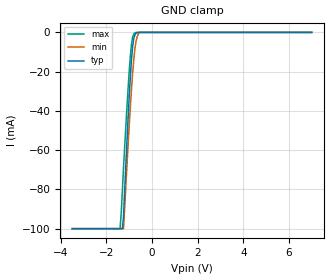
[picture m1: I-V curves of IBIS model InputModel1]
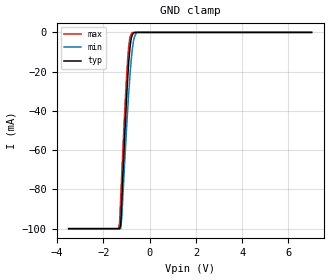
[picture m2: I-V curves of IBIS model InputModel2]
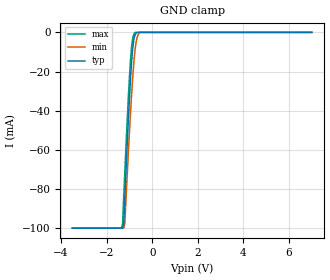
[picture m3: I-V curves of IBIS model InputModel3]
[IBIS Ver]   2.1
[File name]   e_002bl3.ibs   | e_= TSOP, f002bl= abbr chip name, 3= 3.3V Vcc
[File Rev]   2.00
[Date]   13-March-1996
[Source]   File generated from lab measurements at Intel Corporation
[Notes]   Rev 2.00 All data was replaced by actual measurements
   performed in a lab.
[Disclaimer] INTEL DEVELOPER'S SOFTWARE LICENSE AGREEMENT
| BY USING THIS SOFTWARE, YOU ARE AGREEING TO BE BOUND
| BY THE TERMS OFTHIS AGREEMENT.  DO NOT USE THE SOFTWARE
| UNTIL YOU HAVE CAREFULLY READAND AGREED TO THE FOLLOWING
| TERMS AND CONDITIONS.  IF YOU DO NOT AGREETO THE TERMS
| OF THIS AGREEMENT, PROMPTLY RETURN THE SOFTWARE PACKAGE
| ANDANY ACCOMPANYING ITEMS.
| IF YOU USE THIS SOFTWARE, YOU WILL BE BOUND BY THE TERMS
| OF THIS AGREEMENT
| LICENSE: Intel Corporation ("Intel") grants you the non-exclusive right
| to use the enclosed software program ("Software").  You will not use,
| copy, modify, rent, sell or transfer the Software or any portion
| thereof, except as provided in this Agreement.
| System OEM Developers may:
| 1.   Copy the Software for support, backup or archival purposes;
| 2.   Install, use, or distribute Intel owned Software in object code
|   only;
| 3.   Modify and/or use Software source code that Intel directly makes
|   available to you as an OEM Developer;
| 4.   Install, use, modify, distribute, and/or make or have made
|   derivatives ("Derivatives") of Intel owned Software under the
|   terms and conditions in this Agreement, ONLY if you are a System
|   OEM Developer and NOT an end-user.
| RESTRICTIONS:
| YOU WILL NOT:
| 1.   Copy the Software, in whole or in part, except as provided for
|   in this Agreement;
| 2.   Decompile or reverse engineer any Software provided in object
|   code format;
| 3.   Distribute any Software or Derivative code to any end-users,
|   unless approved by Intel in a prior writing.
| TRANSFER: You may transfer the Software to another OEM
| Developer if thereceiving party agrees to the terms of this
| Agreement at the sole risk of any receiving party.
| OWNERSHIP AND COPYRIGHT OF SOFTWARE:
| Title to the Software and all copies thereof remain with Intel
| or its vendors.  The Software iscopyrighted and is protected by
| United States and international copyright laws.  You will not
| remove the copyright notice from the Software.  You agree to
| prevent any unauthorized copying of the Software.
| DERIVATIVE WORK: OEM Developers that make or have made
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[Copyright]   Copyright 1996, Intel Corporation, All Rights Reserved
[Component]   E28F002BL   | 40-lead TSOP package, 28F002BL
[Manufacturer]  Intel   | Boot Block (tm)
|   | operating in 3.3V Vcc range
[Package]
| The following values apply for the Alloy-42 leadframe.
|Variable   typ   min   max
R_pkg   135m   126m   144m
L_pkg   3.95nH   3.62nH   4.28nH
C_pkg   0.39pF   0.38pF   0.40pF
|***********************Pin Definition********************************
[Pin]   signal_name   model_name   R_pin   L_pin   C_pin
  1   A16   InputModel2
  2   A15   InputModel1
  3   A14   InputModel1
  4   A13   InputModel1
  5   A12   InputModel1
  6   A11   InputModel1
  7   A9   InputModel1
  8   A8   InputModel1
  9   WE#   InputModel5
 10   RP#   InputModel3
 11   VPP   POWER
 12   DU   InputModel6
 13   NC   InputModel1
 14   A7   InputModel1
 15   A6   InputModel1
 16   A5   InputModel1
 17   A4   InputModel1
 18   A3   InputModel1
 19   A2   InputModel1
 20   A1   InputModel1
 21   A0   InputModel2
 22   CE#   InputModel2
 23   GND   GND
 24   OE#   InputModel4
 25   DQ0   InputOutput
 26   DQ1   InputOutput
 27   DQ2   InputOutput
 28   DQ3   InputOutput
 29   NC   InputModel2
 30   VCC   POWER
 31   VCC   POWER
 32   DQ4   InputOutput
 33   DQ5   InputOutput
 34   DQ6   InputOutput
 35   DQ7   InputOutput
 36   A10   InputModel1
 37   NC   InputModel6
 38   NC   InputModel6
 39   GND   GND
 40   A17   InputModel1
|***********************Input Model 6******************************
[Model]   InputModel6
Model_type   Input
|   Model for  DU & NC pins, excluding Pin #13.
Vinl = 0.8V
Vinh = 2.0V
|Variable   Typ   Min   Max
C_comp   5.61p   NA   7.6p
[Voltage Range]   3.3V   3.0V   3.6V
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| Models and submodels in the file (7): InputModel1 (Input), InputModel2 (Input), InputModel3 (Input), InputModel4 (Input), InputModel5 (Input), InputModel6 (Input), InputOutput (I/O)
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|*********************Input Model 1************************************
[Model]   InputModel1
Model_type   Input
|   Model for A[15:1] A[17] & NC (pin 13).
Vinl = 0.8V
Vinh = 2.0V
|Variable   Typ   Min   Max
C_comp   5.61p   NA   7.6p
[Voltage Range]   3.3V   3.0V   3.6V
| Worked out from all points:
|   GND clamp passes 1 mA (typ) near -0.74 V on its own axis
[GND_clamp]
|Voltage  I(typ)   I(min)   I(max)
-3.5V     -100mA     -100mA     -100mA
-1.4V     -100mA     -100mA     -100mA
-1.35V    -100mA     -100mA     -92.06mA
-1.3V     -100mA     -100mA     -81.04mA
-1.25V    -94.05mA   -100mA     -69.23mA
-1.1V     -55.84mA   -68.26mA   -38.39mA
-1V       -32.84mA   -47.78mA   -19.9mA
-900mV    -13.97mA   -29.09mA   -6.016mA
-800mV    -3.185mA   -14.07mA   -792.3uA
-700mV    -426.8uA   -4.481mA   0A
-550mV    0A         0A         0A
7V        0A         0A         0A
[Power_clamp]
| Input buffer circuits of this product do not intrinsically
| require a [Power_clamp] definition.  This zero current
| [Power_clamp] table is provided for the compatibility with
| some IBIS parsers.
|Voltage  I(typ)   I(min)   I(max)
-3.3V     0A         0A         0A
0V        0A         0A         0A
3.3V      0A         0A         0A
7V        0A         0A         0A
|*********************Input Model 2******************************
[Model]   InputModel2
Model_type   Input
|   Model for A[0], A[16] & CE# pins.
Vinl = 0.8V
Vinh = 2.0V
|Variable   Typ   Min   Max
C_comp   5.61p   NA   7.6p
[Voltage Range]   3.3V   3.0V   3.6V
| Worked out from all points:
|   GND clamp passes 1 mA (typ) near -0.74 V on its own axis
[GND_clamp]
|Voltage  I(typ)   I(min)   I(max)
-3.5V     -100mA     -100mA     -100mA
-1.35V    -100mA     -100mA     -100mA
-1.3V     -100mA     -100mA     -97.31mA
-1.25V    -97.98mA   -100mA     -83.77mA
-1.2V     -84.29mA   -93.56mA   -70.52mA
-1.05V    -45.71mA   -60.05mA   -33.65mA
-950mV    -23.43mA   -39.44mA   -13.59mA
-850mV    -7.586mA   -21.73mA   -2.468mA
-750mV    -1.17mA    -8.517mA   0A
-650mV    0A         -2.085mA   0A
-550mV    0A         0A         0A
7V        0A         0A         0A
[Power_clamp]
| Input buffer circuits of this product do not intrinsically
| require a [Power_clamp] definition.  This zero current
| [Power_clamp] table is provided for the compatibility with
| some IBIS parsers.
|Voltage  I(typ)   I(min)   I(max)
-3.3V     0A         0A         0A
0V        0A         0A         0A
3.3V      0A         0A         0A
7V        0A         0A         0A
|***********************Input Model 3******************************
[Model]   InputModel3
Model_type   Input
|   Model for RP# pin.
Vinl = 0.8V
Vinh = 2.0V
|Variable   Typ   Min   Max
C_comp   5.61p   NA   7.6p
[Voltage Range]   3.3V   3.0V   3.6V
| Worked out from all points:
|   GND clamp passes 1 mA (typ) near -0.74 V on its own axis
[GND_clamp]
|Voltage  I(typ)   I(min)   I(max)
-3.5V     -100mA     -100mA     -100mA
-1.35V    -100mA     -100mA     -100mA
-1.3V     -100mA     -100mA     -97.77mA
-1.25V    -97.89mA   -100mA     -84.11mA
-1.2V     -84.17mA   -97.43mA   -70.88mA
-1.05V    -45.52mA   -62.23mA   -33.85mA
-950mV    -23.27mA   -40.65mA   -13.74mA
-850mV    -7.538mA   -22.21mA   -2.542mA
-750mV    -1.177mA   -8.633mA   0A
-650mV    0A         -2.115mA   0A
-550mV    0A         0A         0A
7V        0A         0A         0A
[Power_clamp]
| Input buffer circuits of this product do not intrinsically
| require a [Power_clamp] definition.  This zero current
| [Power_clamp] table is provided for the compatibility with
| some IBIS parsers.
|Voltage  I(typ)   I(min)   I(max)
-3.3V     0A         0A         0A
0V        0A         0A         0A
3.3V      0A         0A         0A
7V        0A         0A         0A
